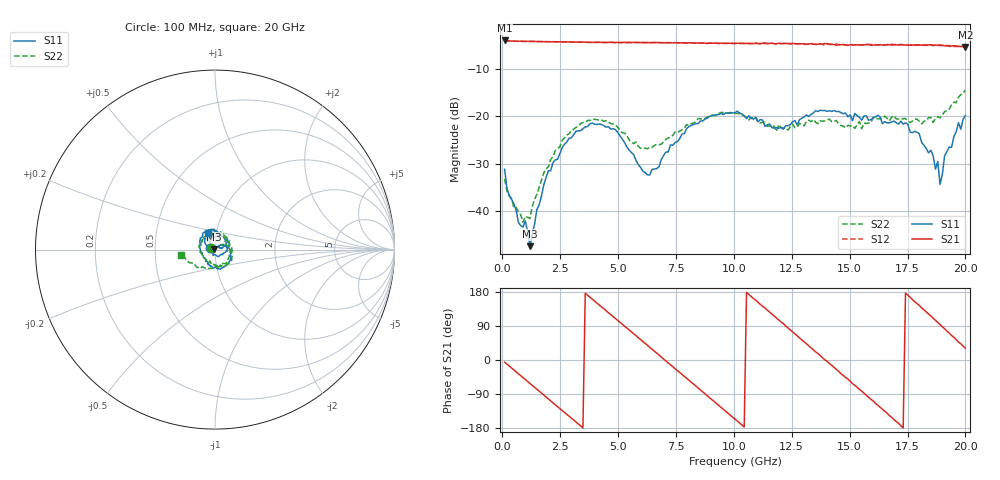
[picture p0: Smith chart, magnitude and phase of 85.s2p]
!Agilent Technologies,N5230C,MY49001569,A.09.33.09
!Agilent N5230C: A.09.33.09
!Date: Tuesday, July 28, 2015 17:45:41
!Correction: S11(Full 2 Port(1,2))
!S21(Full 2 Port(1,2))
!S12(Full 2 Port(1,2))
!S22(Full 2 Port(1,2))
!S2P File: Measurements: S11, S21, S12, S22:
# Hz S  dB  R 50
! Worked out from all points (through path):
!   201 points, 100 MHz to 20 GHz, reference 50 ohm
!   highest |S21| = -3.99 dB at 100 MHz (marker M1); lowest = -5.3 dB at 20 GHz (marker M2)
!   group delay of S21, straight-line fit = 145 ps
!   lowest |S11| = -47.3 dB at 1.194 GHz (marker M3), VSWR 1.01, Z = 49.6 + j0.184 ohm
!   |S11| at or under -10 dB: start of sweep to end of sweep
!   |S22| runs from -42.3 to -14.5 dB; largest |S21 - S12| = 0.025
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1e8  -31.12 160.3  -3.99 -5.9  -4.02 -5.7  -33.17 152.8
8.96e8  -43.29 136.8  -4.20 -46.5  -4.16 -46.6  -42.29 163.5
1.1945e9  -47.32 154.5  -4.18 -61.7  -4.21 -61.9  -41.49 179.6
1.9905e9  -31.46 154.9  -4.24 -102.7  -4.30 -102.8  -30.64 165.8
3.483e9  -22.59 84.7  -4.34 -178.9  -4.35 -179.1  -21.29 101.3
5.274e9  -25.46 20.4  -4.38 89.7  -4.42 89.5  -23.48 36.4
6.269e9  -32.31 39.3  -4.40 38.7  -4.47 38.6  -26.80 33.9
6.7665e9  -30.62 44.0  -4.44 13.1  -4.44 12.9  -25.95 35.1
7.5625e9  -25.31 26.3  -4.47 -27.9  -4.50 -28.3  -23.40 19.8
8.5575e9  -20.92 -13.0  -4.55 -79.2  -4.52 -79.4  -20.52 -6.1
1.005e10  -19.23 -72.1  -4.59 -156.3  -4.66 -156.1  -19.38 -51.3
1.09455e10  -20.29 -105.1  -4.62 157.9  -4.49 156.7  -20.13 -77.1
1.19405e10  -22.49 -156.6  -4.57 105.5  -4.63 105.1  -21.71 -117.0
1.3433e10  -19.29 129.2  -4.79 27.1  -4.73 26.8  -20.65 158.0
1.4428e10  -18.98 98.3  -4.99 -24.9  -4.71 -24.3  -20.85 123.0
1.53235e10  -19.84 85.5  -4.89 -71.8  -4.92 -72.0  -21.76 114.0
1.67165e10  -21.35 51.7  -4.90 -146.5  -4.76 -145.7  -20.91 70.2
1.801e10  -23.64 -9.0  -4.91 143.9  -5.02 143.0  -21.02 -8.9
1.8806e10  -29.47 -109.2  -5.04 99.3  -4.84 98.6  -20.02 -81.7
1.89055e10  -34.30 -122.3  -4.97 93.4  -5.11 93.3  -20.29 -86.4
1.91045e10  -28.23 -167.7  -5.08 82.3  -5.10 81.8  -18.99 -110.7
2e10  -19.81 113.5  -5.35 31.2  -5.36 31.1  -14.45 -171.7
